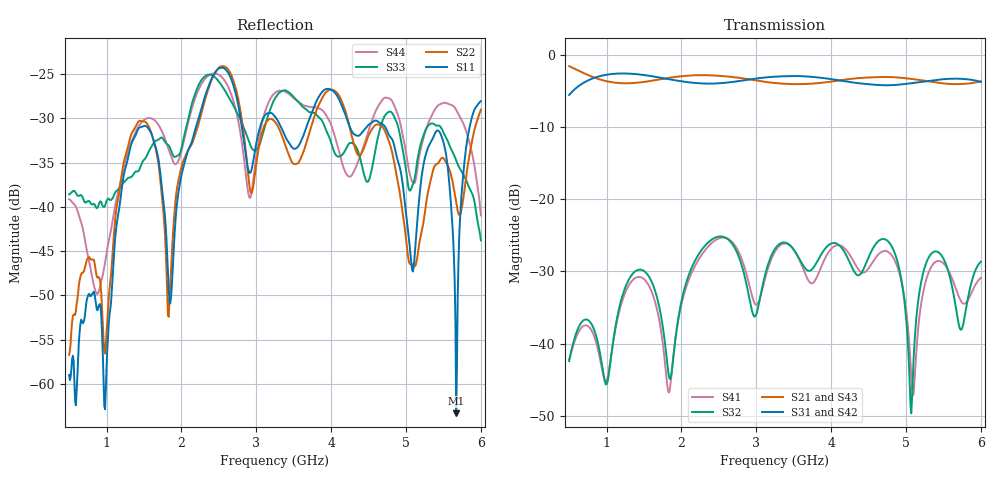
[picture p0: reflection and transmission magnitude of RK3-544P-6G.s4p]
! MTS Systemtechnik GmbH
! S-Parameters
! Model: RK3-544P-6G
! Rohde & Schwarz ZVB8 2Ports - Version 3.20 - 1145.1010k08 SN: 100119
! Converted & adapted with Octave
!  | 	MTS  |
!  IN (Port 1) o--|  |--o -3dB / 0° (Port 2)
!  | RK3-544P-6G |
! ISO (Port 4) o--|		|--o -3dB / 90° (Port 3)
! S4P File: Measurements:
! <S11,S12,S13,S14>,
! <S21,S22,S23,S24>,
! <S31,S32,S33,S34>,
! <S41,S42,S43,S44>:
# HZ  S  DB  R  50.00
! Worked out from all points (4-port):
!   551 points, 500 MHz to 6 GHz, reference 50 ohm
!   strongest paths, dB at 500 MHz, 1.87 GHz, 3.25 GHz, 4.63 GHz, 6 GHz:
!     S31: -5.5, -3.4, -3.0, -4.2, -3.7
!     S42: -5.5, -3.4, -3.0, -4.2, -3.7
!     S21: -1.6, -3.1, -3.9, -3.1, -3.6
!     S43: -1.6, -3.1, -3.9, -3.1, -3.6
!     S32: -42.4, -43.9, -26.9, -25.8, -28.7
!     S41: -42.2, -44.0, -27.2, -27.6, -30.9
!   lowest |S11| = -63.3 dB at 5.67 GHz (marker M1), VSWR 1.00, Z = 50 - j0.067 ohm
!   |S11| at or under -10 dB: start of sweep to end of sweep
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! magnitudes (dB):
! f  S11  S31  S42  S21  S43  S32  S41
! 500 MHz  -59.0  -5.5  -5.5  -1.6  -1.6  -42.4  -42.2
! 2.53 GHz  -24.3  -3.9  -3.9  -2.9  -2.9  -25.1  -25.3
! 4.75 GHz  -31.5  -4.2  -4.2  -3.1  -3.1  -25.7  -27.2
! 5.07 GHz  -46.3  -3.9  -3.9  -3.3  -3.3  -49.6  -44.2
! 5.44 GHz  -31.5  -3.4  -3.4  -3.9  -3.9  -27.4  -28.5
! 5.67 GHz  -63.3  -3.3  -3.3  -4.0  -4.1  -35.3  -32.5
! 6 GHz  -28.1  -3.7  -3.7  -3.6  -3.6  -28.7  -30.9
